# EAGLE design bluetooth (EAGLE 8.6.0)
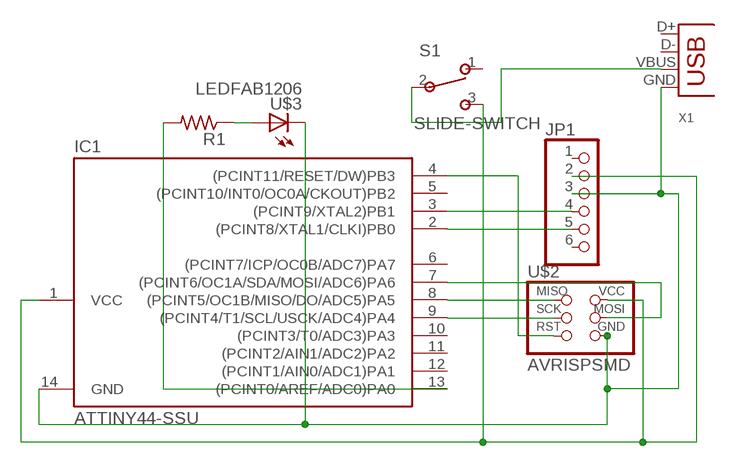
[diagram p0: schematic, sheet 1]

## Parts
IC1  ATTINY44-SSU  [SOIC14]
JP1  PINHD-1X6  [1X06]
R1  RES-US1206FAB  [R1206FAB]
S1  SLIDE-SWITCH  [AYZ0102AGRLC]
U$2  AVRISPSMD  [2X03SMD]
U$3  LEDFAB1206  [LED1206FAB]
X1  USB-A-S  [USB-A-S]

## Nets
N$1: IC1.8((PCINT5/OC1B/MISO/DO/ADC5)PA5) U$2.1(MISO)
N$2: IC1.9((PCINT4/T1/SCL/USCK/ADC4)PA4) U$2.3(SCK)
N$3: IC1.7((PCINT6/OC1A/SDA/MOSI/ADC6)PA6) U$2.4(MOSI)
N$4: IC1.1(VCC) JP1.2 S1.3 U$2.2(VCC)
N$5: IC1.14(GND) JP1.3 U$2.6(GND) U$3.2(C) X1.GND
N$6: IC1.4((PCINT11/RESET/DW)PB3) U$2.5(RST)
N$7: IC1.2((PCINT8/XTAL1/CLKI)PB0) JP1.5
N$8: IC1.3((PCINT9/XTAL2)PB1) JP1.4
N$9: R1.1 U$3.1(A)
N$10: IC1.13((PCINT0/AREF/ADC0)PA0) R1.2
N$11: S1.2 X1.VBUS
Unconnected: IC1.5((PCINT10/INT0/OC0A/CKOUT)PB2) IC1.6((PCINT7/ICP/OC0B/ADC7)PA7) IC1.10((PCINT3/T0/ADC3)PA3) IC1.11((PCINT2/AIN1/ADC2)PA2) IC1.12((PCINT1/AIN0/ADC1)PA1) JP1.1 JP1.6 S1.1 X1.D+ X1.D-

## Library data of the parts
IC1 = fab:ATTINY44
JP1 = pinhead:PINHD-1X6: PIN HEADER
R1 = fab:RES-US: Resistor (US Symbol)
S1 = fab:SLIDE-SWITCH: SMD slide-switch AYZ0102AGRLC as found in the fablab inventory. Includes the mounting holes. Made by Zaerc.
U$2 = fab:AVRISP
U$3 = fab:LED: LED
X1 = con-usb-3:USB: USB Connectors

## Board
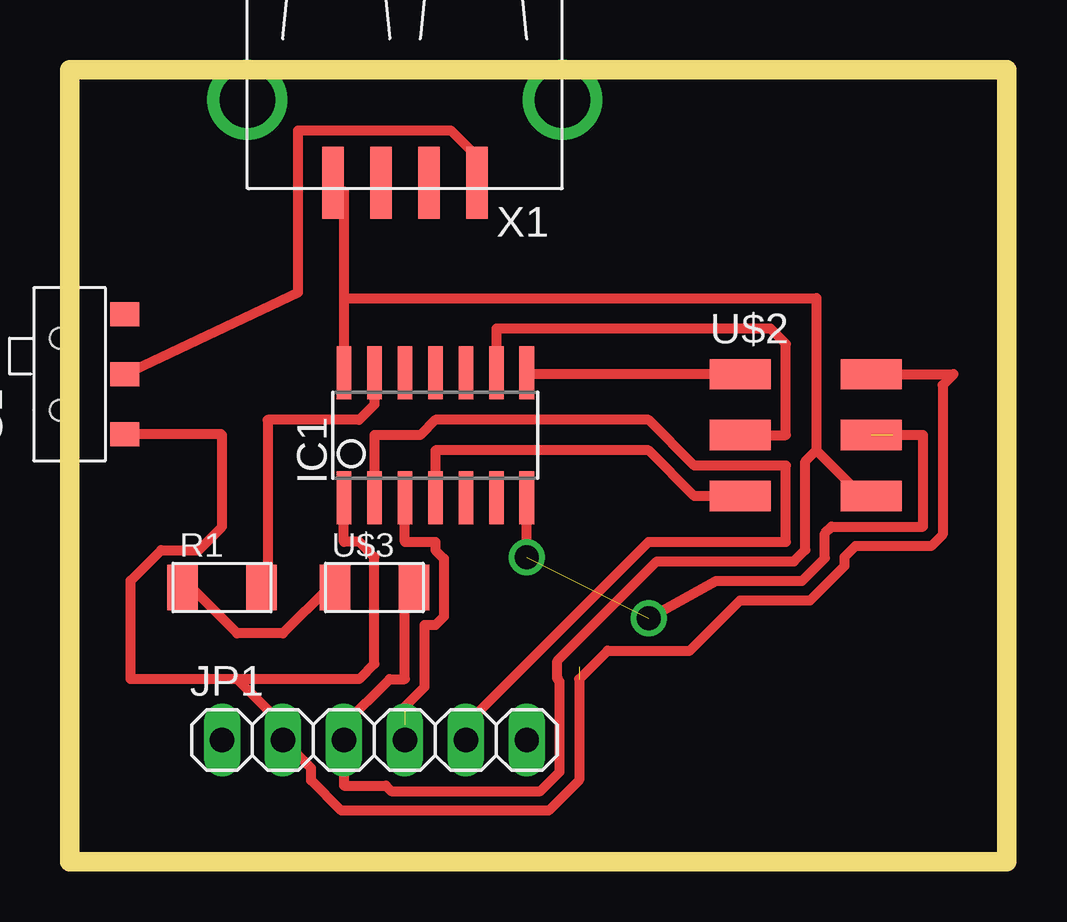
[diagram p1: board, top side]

Size 39.04 x 33.01 mm. Coordinates in mm from the lower left corner, seen from the top.
Outline: 0,0 39.04,0 39.04,33.01 0,33.01 0,0
Copper layers (1*16): Top 0.035mm / dielectric 1.5mm / Bottom 0.035mm
Design rules "default *": minimum track width 16mil, minimum drill 0.35mm, track to track 16mil, track to pad 16mil, pad to pad 16mil, via to via 16mil, smd to smd 16mil, copper to edge 16mil, drill to drill 16mil, minimum pad ring 10mil, minimum via ring 8mil, stop-mask expansion 4mil, vias tented up to drill 0mil, thermal gap 10mil

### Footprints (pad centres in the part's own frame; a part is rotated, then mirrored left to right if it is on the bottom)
SOIC14 = smd 0.61 x 2.21: 1 -3.81,-2.603; 2 -2.54,-2.603; 3 -1.27,-2.603; 4 0,-2.603; 5 1.27,-2.603; 6 2.54,-2.603; 7 3.81,-2.603; 8 3.81,2.603; 9 2.54,2.603; 10 1.27,2.603; 11 0,2.603; 12 -1.27,2.603; 13 -2.54,2.603; 14 -3.81,2.603
1X06 = drill 1.016 long: 1 -6.35,0; 2 -3.81,0; 3 -1.27,0; 4 1.27,0; 5 3.81,0; 6 6.35,0
R1206FAB = smd 1.27 x 1.905: 1 -1.651,0; 2 1.651,0
AYZ0102AGRLC = smd 1 x 1.2: 1 2.5,-2.3; 2 0,-2.3; 3 -2.5,-2.3 | hole 0.85: -1.5,0.4; 1.5,0.4
2X03SMD = smd 2.54 x 1.27: 1 -2.54,2.54; 2 2.92,2.54; 3 -2.54,0; 4 2.92,0; 5 -2.54,-2.54; 6 2.92,-2.54
LED1206FAB = smd 1.27 x 1.905: 1 -1.651,0; 2 1.651,0
USB-A-S = smd 3 x 0.9: D+ 3.45,-1; D- 3.45,1; GND 3.45,-3; VBUS 3.45,3 | drill 2.311: P$5 0,-6.566; P$6 0,6.566

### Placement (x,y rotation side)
IC1  15.24,17.78 0 top
JP1  12.7,5.08 0 top
R1  6.35,11.43 0 top
S1  0,20.32 90 top
U$2  30.48,17.78 0 top
U$3  12.7,11.43 0 top
X1  13.97,31.75 270 top

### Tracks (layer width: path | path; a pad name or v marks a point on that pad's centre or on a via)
N$1
  Top 0.406: U$2.1 19.05,20.32 IC1.8
N$2
  Top 0.406: IC1.9 17.78,22.22 29.21,22.22 29.84,21.59 29.84,17.78 U$2.3
N$3  (via drill 1)  (2 unrouted)
  Top 0.406: v19.05,12.7 IC1.7 | v24.13,10.16 26.95,11.71 30.52,11.71 31.47,12.66 31.47,13.69 31.75,13.97 35.56,13.97 35.56,17.78 34.29,17.78
N$4  (1 unrouted)
  Top 0.406: 6.98,7.62 8.89,5.71 JP1.2 10.06,3.91 10.06,3.4 11.32,2.13 19.95,2.13 21.23,3.41 21.23,7.62 22.41,8.8 25.84,8.8 27.94,10.9 30.85,10.9 32.28,12.32 32.28,12.7 32.74,13.16 35.9,13.16 36.37,13.63 36.37,19.86 36.83,20.32 U$2.2 33.66,20.32 | IC1.1 11.43,13.33 12.06,13.33 12.7,12.7 12.7,8.25 12.06,7.62 6.98,7.62 | 6.98,7.62 2.54,7.62 2.54,11.72 3.81,12.99 5.37,12.99 6.35,13.97 6.35,17.78 6.31,17.82 S1.3
N$5
  Top 0.406: U$3.2 13.97,11.43 13.97,7.62 13.34,7.62 11.43,5.71 JP1.3 11.43,3.17 13.17,3.17 13.4,2.95 19.62,2.95 20.42,3.75 20.42,7.52 20.32,7.62 20.32,8.38 24.47,12.52 30.18,12.52 30.66,13 30.66,16.69 31.12,17.14 | 11.43,23.5 11.43,27.94 10.8,27.94 X1.GND | 11.43,23.5 IC1.14 | 31.12,17.14 33.02,15.24 U$2.6 | 31.12,17.14 31.12,23.5 11.43,23.5
N$6
  Top 0.406: IC1.4 15.24,17.14 24.13,17.14 26.03,15.24 U$2.5
N$7
  Top 0.406: IC1.2 12.7,17.78 14.6,17.78 15.24,18.41 24.13,18.41 26.03,16.51 29.84,16.51 29.84,13.33 24.13,13.33 16.51,5.71 JP1.5
N$8  (1 unrouted)
  Top 0.406: IC1.3 13.97,13.33 15.24,13.33 15.24,12.99 15.6,12.64 15.6,10.22 15.24,9.87 14.78,9.87 14.78,7.28 13.97,6.47 13.97,6.35 | JP1.4 13.97,5.71
N$9
  Top 0.406: R1.1 5.08,11.43 6.98,9.53 8.89,9.53 10.8,11.43 U$3.1
N$10
  Top 0.406: IC1.13 12.7,19.05 12.06,18.41 8.26,18.41 8.26,11.43 R1.2
N$11
  Top 0.406: X1.VBUS 17.15,28.57 17.15,29.21 15.88,30.48 9.52,30.48 9.52,23.73 S1.2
